| IBIS file stm32l4p5_4q5_lqfp48.ibs
[IBIS ver]   4.2
[File name]  stm32l4p5_4q5_lqfp48.ibs
[File Rev]   1.0
[Date]   04-10-2019
[Source]   Data Created at STMicroelectronics
[Notes]   File originated from ELDO simulations.
[Disclaimer] This information is for modeling purpose only and is
   not guaranted.
   The information is subject to change without notice.
[Copyright]  Copyright 2019 STMicroelectronics Inc.
|   Component stm32l4p5_4q5_lqfp48
[Component] stm32l4p5_4q5_lqfp48
[Manufacturer] STMicroelectronics
[Package]
| variable   typ   min   max
R_pkg  0  NA  NA
L_pkg  0  NA  NA
C_pkg  0  NA  NA
[Pin]   signal_name   model_name R_pin L_pin C_pin
1 VBAT POWER 0.053 3.42534E-09 9.041E-14
2 PC13 io8prog2m25m50m120m_sudq_ft 0.048377332 2.91404E-09 6.443E-14
3 PC14-OSC32_IN io8prog2m25m50m120m_sudq_ft 0.044678997 2.50442E-09 4.365E-14
4 PC15-OSC32_OUT io8prog2m25m50m120m_sudq_ft 0.041905328 2.19704E-09 2.807E-14
5 PH0-OSC_IN io8prog2m25m50m120m_sudq_ft 0.040056325 1.9919E-09 1.769E-14
6 PH1-OSC_OUT io8prog2m25m50m120m_sudq_ft 0.03913 1.89021E-09 1.24625E-14
7 NRST ioreset_ft_v33 0.03913 1.89021E-09 1.24625E-14
8 VSSA GND 0.040057312 1.98992E-09 1.775E-14
9 VDDA POWER 0.041906973 2.19374E-09 2.817E-14
10 PA0 io8prog2m25m50m120m_sudq_ft 0.0446813 2.4998E-09 4.379E-14
11 PA1 io8prog2m25m50m120m_sudq_ft 0.048380293 2.9081E-09 6.461E-14
12 PA2 io8prog2m25m50m120m_sudq_ft 0.053 3.42534E-09 9.041E-14
13 PA3 io8prog2m25m50m120m_sudq_ft 0.053 3.42534E-09 9.041E-14
14 PA4 io8prog2m25m50m120m_sudq_ft 0.048377332 2.91404E-09 6.443E-14
15 PA5 io8prog2m25m50m120m_sudq_ft 0.044678997 2.50442E-09 4.365E-14
16 PA6 io8prog2m25m50m120m_sudq_ft 0.041905328 2.19704E-09 2.807E-14
17 PA7 io8prog2m25m50m120m_sudq_ft 0.040056325 1.9919E-09 1.769E-14
18 PB0 io8prog2m25m50m120m_sudq_ft 0.03913 1.89021E-09 1.24625E-14
19 PB1 io8prog2m25m50m120m_sudq_ft 0.03913 1.89021E-09 1.24625E-14
20 PB2 io8prog2m25m50m120m_sudq_ft 0.040057312 1.98992E-09 1.775E-14
21 PB10 io8prog2m25m50m120m_sudq_i2c_ft 0.041906973 2.19374E-09 2.817E-14
22 PB11 io8prog2m25m50m120m_sudq_i2c_ft 0.0446813 2.4998E-09 4.379E-14
23 VSS GND 0.048380293 2.9081E-09 6.461E-14
24 VDD POWER 0.053 3.42534E-09 9.041E-14
25 PB12 io8w_swp_lcd4_ft 0.053 3.42534E-09 9.041E-14
26 PB13 io8prog2m25m50m120m_sudq_i2c_ft 0.048377332 2.91404E-09 6.443E-14
27 PB14 io8prog2m25m50m120m_sudq_i2c_ft 0.044678997 2.50442E-09 4.365E-14
28 PB15 io8prog2m25m50m120m_sudq_ft 0.041905328 2.19704E-09 2.807E-14
29 PA8 io8prog2m25m50m120m_sudq_ft 0.040056325 1.9919E-09 1.769E-14
30 PA9 POWER 0.03913 1.89021E-09 1.24625E-14
31 PA10 io8usb_id_otg20_lcd4_ft_ms 0.03913 1.89021E-09 1.24625E-14
32 PA11 io8usblsfs_otg2 0.040057312 1.98992E-09 1.775E-14
33 PA12 io8usblsfs_otg2 0.041906973 2.19374E-09 2.817E-14
34 PA13 io8prog2m25m50m120m_sudq_ft 0.0446813 2.4998E-09 4.379E-14
35 VSS GND 0.048380293 2.9081E-09 6.461E-14
36 VDDUSB POWER 0.053 3.42534E-09 9.041E-14
37 PA14 io8prog2m25m50m120m_sudq_ft 0.053 3.42534E-09 9.041E-14
38 PA15 io8prog2m25m50m120m_sudq_ft 0.048377332 2.91404E-09 6.443E-14
39 PB3 io8prog2m25m50m120m_sudq_ft 0.044678997 2.50442E-09 4.365E-14
40 PB4 io8prog2m25m50m120m_sudq_ft 0.041905328 2.19704E-09 2.807E-14
41 PB5 io8prog2m25m50m120m_sudq_ft 0.040056325 1.9919E-09 1.769E-14
42 PB6 io8prog2m25m50m120m_sudq_i2c_ft 0.03913 1.89021E-09 1.24625E-14
43 PB7 io8prog2m25m50m120m_sudq_i2c_ft 0.03913 1.89021E-09 1.24625E-14
44 PH3-BOOT0 io8prog2m25m50m120m_sudq_ft 0.040057312 1.98992E-09 1.775E-14
45 PB8 io8prog2m25m50m120m_sudq_i2c_ft 0.041906973 2.19374E-09 2.817E-14
46 PB9 io8prog2m25m50m120m_sudq_i2c_ft 0.0446813 2.4998E-09 4.379E-14
47 VSS GND 0.048380293 2.9081E-09 6.461E-14
48 VDD POWER 0.053 3.42534E-09 9.041E-14
[Model Selector] io8prog2m25m50m120m_sudq_ft
iols8p_sudq_ft_pd_lv  "IO low speed, PD=40kOhm - 1P8V"
iols8p_sudq_ft_pu_lv  "IO low speed, PU=40kOhm - 1P8V"
iols8p_sudq_ft_lv  "IO low speed - 1P8V"
iols8p_sudq_ft_pd  "IO low speed, PD=40kOhm - 3P3V"
iols8p_sudq_ft_pu  "IO low speed, PU=40kOhm - 3P3V"
iols8p_sudq_ft  "IO low speed - 3P3V"
iofs8p_sudq_ft_pd_lv  "IO full speed, PD=40kOhm - 1P8V"
iofs8p_sudq_ft_pu_lv  "IO full speed, PU=40kOhm - 1P8V"
iofs8p_sudq_ft_lv  "IO full speed - 1P8V"
iofs8p_sudq_ft_pd  "IO full speed, PD=40kOhm - 3P3V"
iofs8p_sudq_ft_pu  "IO full speed, PU=40kOhm - 3P3V"
iofs8p_sudq_ft  "IO full speed - 3P3V"
ioms8p_sudq_ft_pd_lv  "IO medium speed, PD=40kOhm - 1P8V"
ioms8p_sudq_ft_pu_lv  "IO medium speed, PU=40kOhm - 1P8V"
ioms8p_sudq_ft_lv  "IO medium speed - 1P8V"
ioms8p_sudq_ft_pd  "IO medium speed, PD=40kOhm - 3P3V"
ioms8p_sudq_ft_pu  "IO medium speed, PU=40kOhm - 3P3V"
ioms8p_sudq_ft  "IO medium speed - 3P3V"
iohs8p_sudq_ft_pd_lv  "IO high speed, PD=40kOhm - 1P8V"
iohs8p_sudq_ft_pu_lv  "IO high speed, PU=40kOhm - 1P8V"
iohs8p_sudq_ft_lv  "IO high speed - 1P8V"
iohs8p_sudq_ft_pd  "IO high speed, PD=40kOhm - 3P3V"
iohs8p_sudq_ft_pu  "IO high speed, PU=40kOhm - 3P3V"
iohs8p_sudq_ft  "IO high speed - 3P3V"
[Model Selector] io8prog2m25m50m120m_sudq_i2c_ft
io8prog_1v8_i2c_pd  "5V Tol GPIO 1.8V range i2c functionality with pull down"
io8prog_1v8_i2c_pu  "5V Tol GPIO 1.8V range i2c functionality with pull up"
io8prog_1v8_i2c  "5V Tol GPIO 1.8V range i2c functionality"
io8prog_3v3_i2c_pd  "5V Tol GPIO 3.3V range i2c functionality with pull down"
io8prog_3v3_i2c_pu  "5V Tol GPIO 3.3V range i2c functionality with pull up"
io8prog_3v3_i2c  "5V Tol GPIO 3.3V range i2c functionality"
iols8p_sudq_ft_pd_lv  "IO low speed, PD=40kOhm - 1P8V"
iols8p_sudq_ft_pu_lv  "IO low speed, PU=40kOhm - 1P8V"
iols8p_sudq_ft_lv  "IO low speed - 1P8V"
iols8p_sudq_ft_pd  "IO low speed, PD=40kOhm - 3P3V"
iols8p_sudq_ft_pu  "IO low speed, PU=40kOhm - 3P3V"
iols8p_sudq_ft  "IO low speed - 3P3V"
iofs8p_sudq_ft_pd_lv  "IO full speed, PD=40kOhm - 1P8V"
iofs8p_sudq_ft_pu_lv  "IO full speed, PU=40kOhm - 1P8V"
iofs8p_sudq_ft_lv  "IO full speed - 1P8V"
iofs8p_sudq_ft_pd  "IO full speed, PD=40kOhm - 3P3V"
iofs8p_sudq_ft_pu  "IO full speed, PU=40kOhm - 3P3V"
iofs8p_sudq_ft  "IO full speed - 3P3V"
ioms8p_sudq_ft_pd_lv  "IO medium speed, PD=40kOhm - 1P8V"
ioms8p_sudq_ft_pu_lv  "IO medium speed, PU=40kOhm - 1P8V"
ioms8p_sudq_ft_lv  "IO medium speed - 1P8V"
ioms8p_sudq_ft_pd  "IO medium speed, PD=40kOhm - 3P3V"
ioms8p_sudq_ft_pu  "IO medium speed, PU=40kOhm - 3P3V"
ioms8p_sudq_ft  "IO medium speed - 3P3V"
iohs8p_sudq_ft_pd_lv  "IO high speed, PD=40kOhm - 1P8V"
iohs8p_sudq_ft_pu_lv  "IO high speed, PU=40kOhm - 1P8V"
iohs8p_sudq_ft_lv  "IO high speed - 1P8V"
iohs8p_sudq_ft_pd  "IO high speed, PD=40kOhm - 3P3V"
iohs8p_sudq_ft_pu  "IO high speed, PU=40kOhm - 3P3V"
iohs8p_sudq_ft  "IO high speed - 3P3V"
[Model Selector] io8w_swp_lcd4_ft
io8w_swp_classc  "Class C swp functionality"
io8w_swp_classb  "Class B swp functionality"
io8lsw_1v8_pd  "GPIO 1.8V range with pd io low speed"
io8lsw_1v8_pu  "GPIO 1.8V range with pu io low speed"
io8lsw_1v8  "GPIO 1.8V range io low speed"
io8lsw_3v3_pd  "GPIO 3.3V range with pd io low speed"
io8lsw_3v3_pu  "GPIO 3.3V range with pu io low speed"
io8lsw_3v3  "GPIO 3.3V range io low speed"
io8fsw_1v8_pd  "GPIO 1.8V range with pd io full speed"
io8fsw_1v8_pu  "GPIO 1.8V range with pu io full speed"
io8fsw_1v8  "GPIO 1.8V range io full speed"
io8fsw_3v3_pd  "GPIO 3.3V range with pd io full speed"
io8fsw_3v3_pu  "GPIO 3.3V range with pu io full speed"
io8fsw_3v3  "GPIO 3.3V range io full speed"
io8msw_1v8_pd  "GPIO 1.8V range with pd io medium speed"
io8msw_1v8_pu  "GPIO 1.8V range with pu io medium speed"
io8msw_1v8  "GPIO 1.8V range io medium speed"
io8msw_3v3_pd  "GPIO 3.3V range with pd io medium speed"
io8msw_3v3_pu  "GPIO 3.3V range with pu io medium speed"
io8msw_3v3  "GPIO 3.3V range io medium speed"
io8hsw_1v8_pd  "GPIO 1.8V range with pd io high speed"
io8hsw_1v8_pu  "GPIO 1.8V range with pu io high speed"
io8hsw_1v8  "GPIO 1.8V range io high speed"
io8hsw_3v3_pd  "GPIO 3.3V range with pd io high speed"
io8hsw_3v3_pu  "GPIO 3.3V range with pu io high speed"
io8hsw_3v3  "GPIO 3.3V range io high speed"
[Model Selector] io8usblsfs_otg2
usb_ls_pd  "USB Low Speed mode - Pull Down"
usb_ls_pu2  "USB Low Speed mode - Pull up 2"
usb_ls_pu  "USB Low Speed mode - Pull up"
usb_fs  "USB Low Speed mode"
usb_fs_pd  "USB Full Speed mode - Pull Down"
usb_fs_pu2  "USB Full Speed mode - Pull up 2"
usb_fs_pu  "USB Full Speed mode - Pull up"
[Model Selector] io8usb_id_otg20_lcd4_ft_ms
io8usbid_1v8_id_pu  "ID 1V8 range with pull up"
io8usbid_3v3_id_pu  "ID 3V3 range with pull up"
io8usbid_1v8_id  "ID 1V8 range"
io8usbid_3v3_id  "ID 3V3 range"
io8lsusbid_1v8_pd  "GPIO 1.8V range with pd io low speed"
io8lsusbid_1v8_pu  "GPIO 1.8V range with pu io low speed"
io8lsusbid_1v8  "GPIO 1.8V range io low speed"
io8lsusbid_3v3_pd  "GPIO 3.3V range with pd io low speed"
io8lsusbid_3v3_pu  "GPIO 3.3V range with pu io low speed"
io8lsusbid_3v3  "GPIO 3.3V range io low speed"
io8fsusbid_1v8_pd  "GPIO 1.8V range with pd io full speed"
io8fsusbid_1v8_pu  "GPIO 1.8V range with pu io full speed"
io8fsusbid_1v8  "GPIO 1.8V range io full speed"
io8fsusbid_3v3_pd  "GPIO 3.3V range with pd io full speed"
io8fsusbid_3v3_pu  "GPIO 3.3V range with pu io full speed"
io8fsusbid_3v3  "GPIO 3.3V range io full speed"
io8msusbid_1v8_pd  "GPIO 1.8V range with pd io medium speed"
io8msusbid_1v8_pu  "GPIO 1.8V range with pu io medium speed"
io8msusbid_1v8  "GPIO 1.8V range io medium speed"
io8msusbid_3v3_pd  "GPIO 3.3V range with pd io medium speed"
io8msusbid_3v3_pu  "GPIO 3.3V range with pu io medium speed"
io8msusbid_3v3  "GPIO 3.3V range io medium speed"
io8hsusbid_1v8_pd  "GPIO 1.8V range with pd io high speed"
io8hsusbid_1v8_pu  "GPIO 1.8V range with pu io high speed"
io8hsusbid_1v8  "GPIO 1.8V range io high speed"
io8hsusbid_3v3_pd  "GPIO 3.3V range with pd io high speed"
io8hsusbid_3v3_pu  "GPIO 3.3V range with pu io high speed"
io8hsusbid_3v3  "GPIO 3.3V range io high speed"
[Model Selector] ioreset_ft_v33
ioreset_1v2_pu  "RESET 1.2V range with PU"
ioreset_1v2  "RESET 1.2V range"
ioreset_1v8_pu  "RESET 1.8V range with PU"
ioreset_1v8  "RESET 1.8V range"
ioreset_3v3_pu  "RESET 3.3V range with PU"
ioreset_3v3  "RESET 3.3V range"
| Models and submodels in the file (97): iols8p_sudq_ft_pd_lv (I/O), iols8p_sudq_ft_pu_lv (I/O), iols8p_sudq_ft_lv (I/O), iols8p_sudq_ft_pd (I/O), iols8p_sudq_ft_pu (I/O), iols8p_sudq_ft (I/O), iofs8p_sudq_ft_pd_lv (I/O), iofs8p_sudq_ft_pu_lv (I/O), iofs8p_sudq_ft_lv (I/O), iofs8p_sudq_ft_pd (I/O), iofs8p_sudq_ft_pu (I/O), iofs8p_sudq_ft (I/O), ioms8p_sudq_ft_pd_lv (I/O), ioms8p_sudq_ft_pu_lv (I/O), ioms8p_sudq_ft_lv (I/O), ioms8p_sudq_ft_pd (I/O), ioms8p_sudq_ft_pu (I/O), ioms8p_sudq_ft (I/O), iohs8p_sudq_ft_pd_lv (I/O), iohs8p_sudq_ft_pu_lv (I/O), iohs8p_sudq_ft_lv (I/O), iohs8p_sudq_ft_pd (I/O), iohs8p_sudq_ft_pu (I/O), iohs8p_sudq_ft (I/O), io8prog_1v8_i2c_pd (I/O_open_drain), io8prog_1v8_i2c_pu (I/O_open_drain), io8prog_1v8_i2c (I/O_open_drain), io8prog_3v3_i2c_pd (I/O_open_drain), io8prog_3v3_i2c_pu (I/O_open_drain), io8prog_3v3_i2c (I/O_open_drain), io8w_swp_classc (I/O), io8w_swp_classb (I/O), io8lsw_1v8_pd (I/O), io8lsw_1v8_pu (I/O), io8lsw_1v8 (I/O), io8lsw_3v3_pd (I/O), io8lsw_3v3_pu (I/O), io8lsw_3v3 (I/O), io8fsw_1v8_pd (I/O), io8fsw_1v8_pu (I/O), io8fsw_1v8 (I/O), io8fsw_3v3_pd (I/O), io8fsw_3v3_pu (I/O), io8fsw_3v3 (I/O), io8msw_1v8_pd (I/O), io8msw_1v8_pu (I/O), io8msw_1v8 (I/O), io8msw_3v3_pd (I/O), io8msw_3v3_pu (I/O), io8msw_3v3 (I/O), io8hsw_1v8_pd (I/O), io8hsw_1v8_pu (I/O), io8hsw_1v8 (I/O), io8hsw_3v3_pd (I/O), io8hsw_3v3_pu (I/O), io8hsw_3v3 (I/O), usb_ls_pd (I/O), usb_ls_pu2 (I/O), usb_ls_pu (I/O), usb_fs (I/O), usb_fs_pd (I/O), usb_fs_pu2 (I/O), usb_fs_pu (I/O), io8usbid_1v8_id_pu (Input), io8usbid_3v3_id_pu (Input), io8usbid_1v8_id (Input), io8usbid_3v3_id (Input), io8lsusbid_1v8_pd (I/O), io8lsusbid_1v8_pu (I/O), io8lsusbid_1v8 (I/O), io8lsusbid_3v3_pd (I/O), io8lsusbid_3v3_pu (I/O), io8lsusbid_3v3 (I/O), io8fsusbid_1v8_pd (I/O), io8fsusbid_1v8_pu (I/O), io8fsusbid_1v8 (I/O), io8fsusbid_3v3_pd (I/O), io8fsusbid_3v3_pu (I/O), io8fsusbid_3v3 (I/O), io8msusbid_1v8_pd (I/O)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
